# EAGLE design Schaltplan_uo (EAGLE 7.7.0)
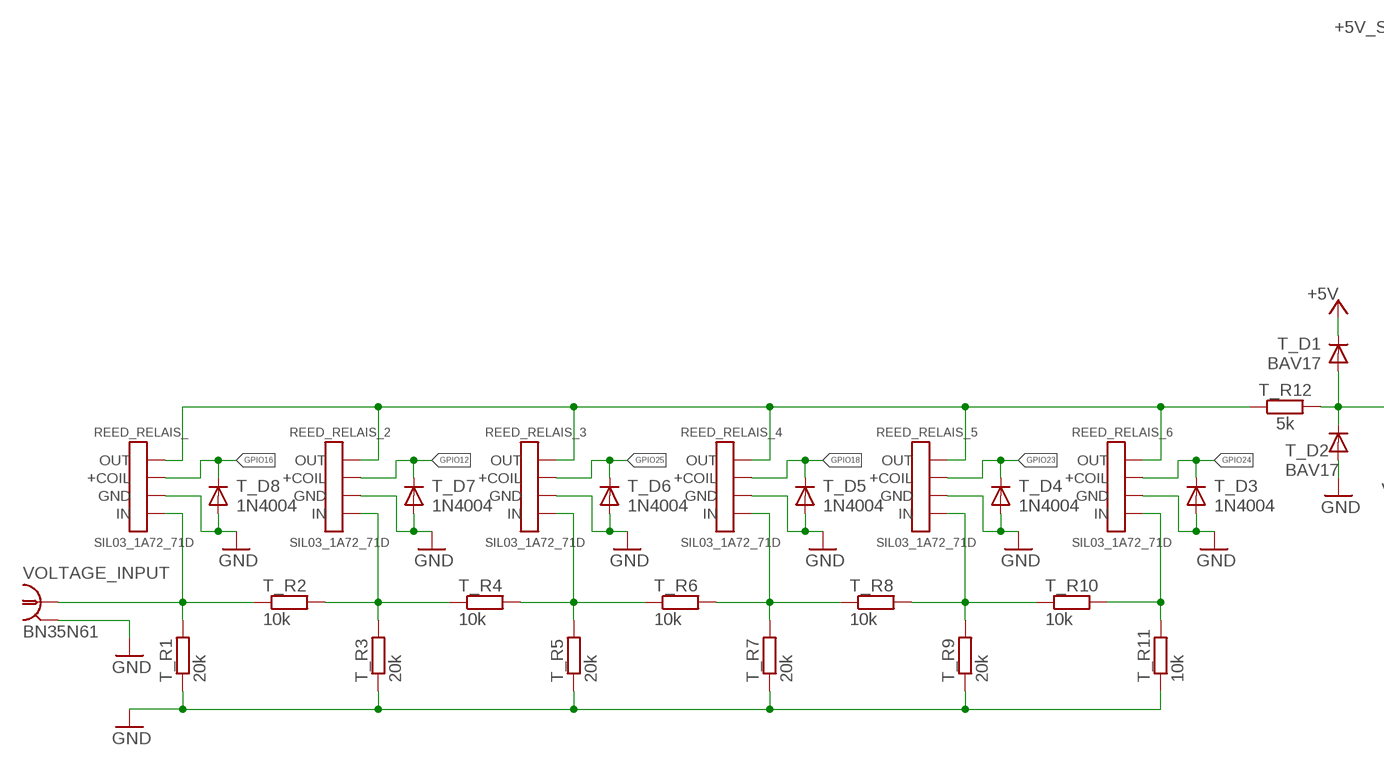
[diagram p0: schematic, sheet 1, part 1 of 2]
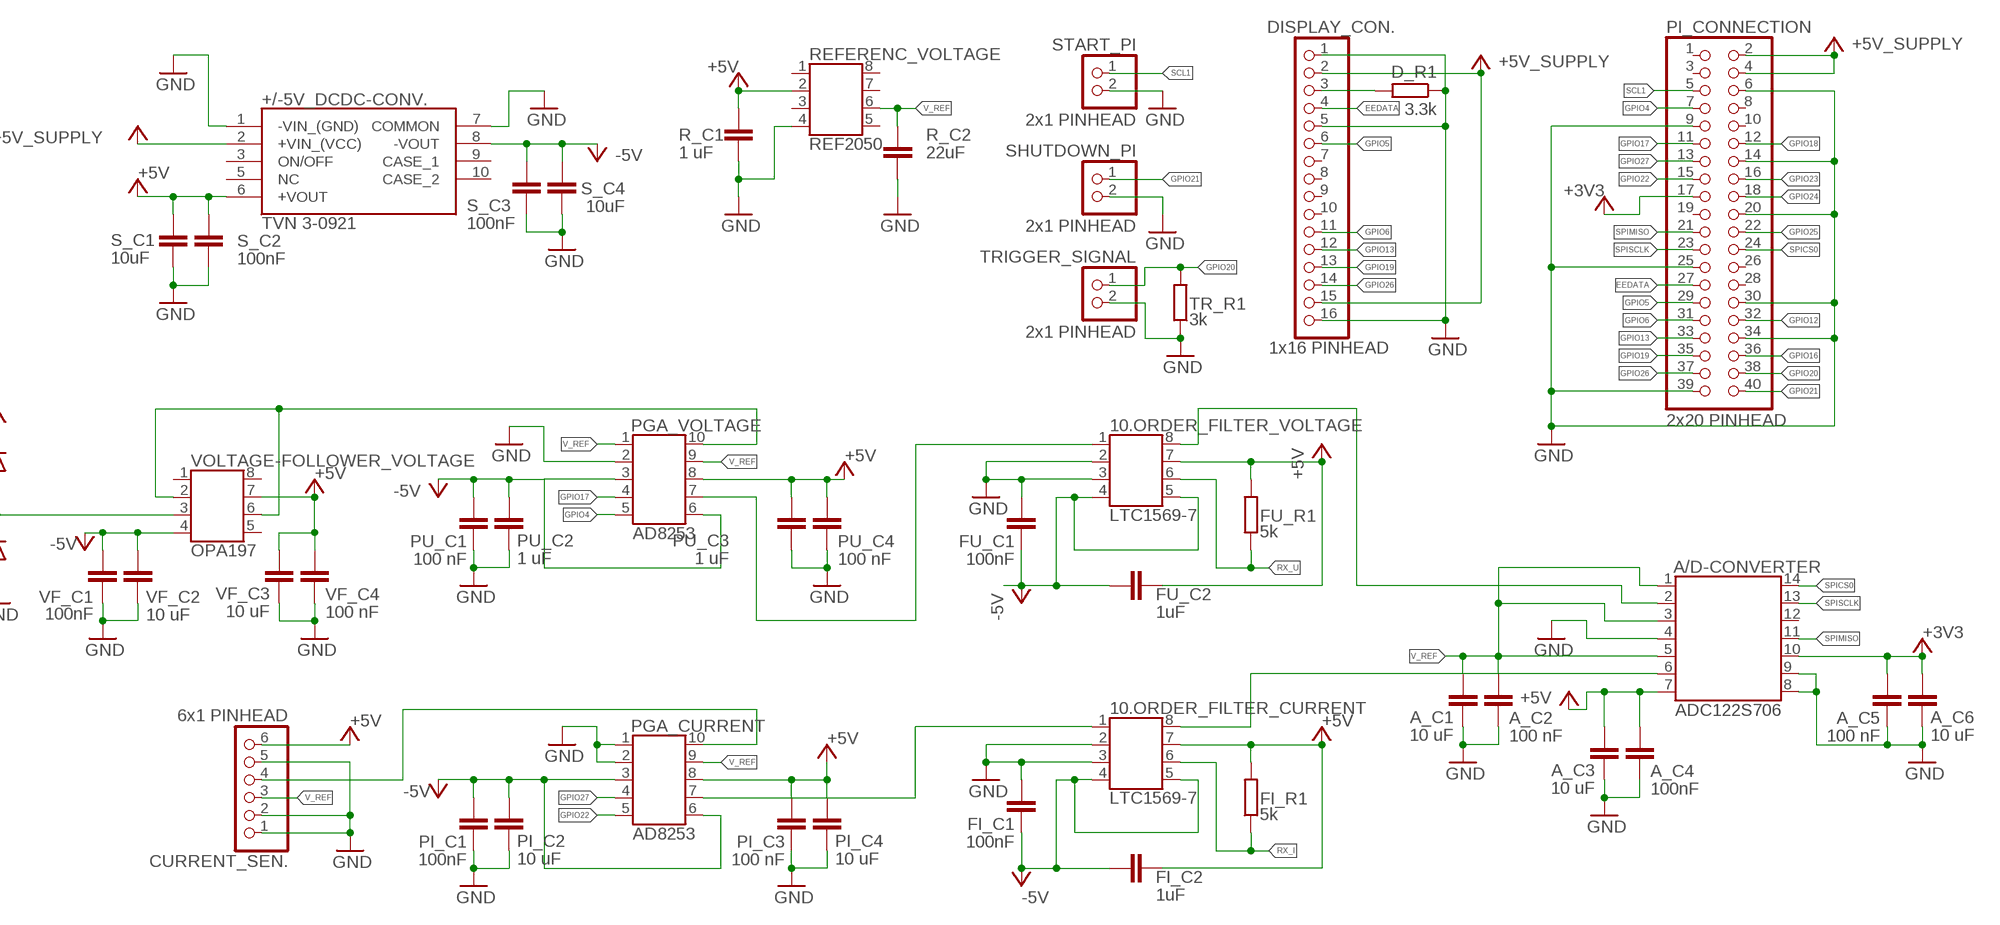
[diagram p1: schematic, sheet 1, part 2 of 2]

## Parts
10.ORDER_FILTER_CURRENT  LTC1569-7  SSOP8_TO_DIP8  [SSOP8_TO_DIP8]
10.ORDER_FILTER_VOLTAGE  LTC1569-7  SSOP8_TO_DIP8  [SSOP8_TO_DIP8]
+/-5V_DCDC-CONV.  TVN 3-0921  TVN_3-1223  [TVN32419]
A/D-CONVERTER  ADC122S706  SSOP14_TO_DIP14-6  [SSOP14_TO_DIP14-6]
A_C1  10 uF  C-EU025-030X050  [C025-030X050]
A_C2  100 nF  C-EU025-030X050  [C025-030X050]
A_C3  10 uF  C-EU025-030X050  [C025-030X050]
A_C4  100nF  C-EU025-030X050  [C025-030X050]
A_C5  100 nF  C-EU025-030X050  [C025-030X050]
A_C6  10 uF  C-EU025-030X050  [C025-030X050]
CURRENT_SEN.  6x1 PINHEAD  PINHD-1X6  [1X06]
D_R1  3.3k  R-EU_0207/10  [0207/10]
DISPLAY_CON.  1x16 PINHEAD  PINHD-1X16  [1X16]
FI_C1  100nF  C-EU025-030X050  [C025-030X050]
FI_C2  1uF  C-EU025-030X050  [C025-030X050]
FI_R1  5k  R-EU_0207/10  [0207/10]
FU_C1  100nF  C-EU025-030X050  [C025-030X050]
FU_C2  1uF  C-EU025-030X050  [C025-030X050]
FU_R1  5k  R-EU_0207/10  [0207/10]
PGA_CURRENT  AD8253  SSOP10_TO_DIP10  [SSOP10_TO_DIP10]
PGA_VOLTAGE  AD8253  SSOP10_TO_DIP10  [SSOP10_TO_DIP10]
PI_C1  100nF  C-EU025-030X050  [C025-030X050]
PI_C2  10 uF  C-EU025-030X050  [C025-030X050]
PI_C3  100 nF  C-EU025-030X050  [C025-030X050]
PI_C4  10 uF  C-EU025-030X050  [C025-030X050]
PI_CONNECTION  2x20 PINHEAD  PINHD-2X20  [2X20]
PU_C1  100 nF  C-EU025-030X050  [C025-030X050]
PU_C2  1 uF  C-EU025-030X050  [C025-030X050]
PU_C3  1 uF  C-EU025-030X050  [C025-030X050]
PU_C4  100 nF  C-EU025-030X050  [C025-030X050]
R_C1  1 uF  C-EU025-030X050  [C025-030X050]
R_C2  22uF  C-EU025-030X050  [C025-030X050]
REED_RELAIS_  SIL03_1A72_71D  REED_REALIS_SIL03_1A72_71D  [REED_RELAIS_SIL03_1A72_71D]
REED_RELAIS_2  SIL03_1A72_71D  REED_REALIS_SIL03_1A72_71D  [REED_RELAIS_SIL03_1A72_71D]
REED_RELAIS_3  SIL03_1A72_71D  REED_REALIS_SIL03_1A72_71D  [REED_RELAIS_SIL03_1A72_71D]
REED_RELAIS_4  SIL03_1A72_71D  REED_REALIS_SIL03_1A72_71D  [REED_RELAIS_SIL03_1A72_71D]
REED_RELAIS_5  SIL03_1A72_71D  REED_REALIS_SIL03_1A72_71D  [REED_RELAIS_SIL03_1A72_71D]
REED_RELAIS_6  SIL03_1A72_71D  REED_REALIS_SIL03_1A72_71D  [REED_RELAIS_SIL03_1A72_71D]
REFERENC_VOLTAGE  REF2050  SSOP8_TO_DIP8  [SSOP8_TO_DIP8]
S_C1  10uF  C-EU025-030X050  [C025-030X050]
S_C2  100nF  C-EU025-030X050  [C025-030X050]
S_C3  100nF  C-EU025-030X050  [C025-030X050]
S_C4  10uF  C-EU025-030X050  [C025-030X050]
SHUTDOWN_PI  2x1 PINHEAD  PINHD-1X2  [1X02]
START_PI  2x1 PINHEAD  PINHD-1X2  [1X02]
T_D1  BAV17  [DO35-10]
T_D2  BAV17  [DO35-10]
T_D3  1N4004  BAV17  [DO35-10]
T_D4  1N4004  BAV17  [DO35-10]
T_D5  1N4004  BAV17  [DO35-10]
T_D6  1N4004  BAV17  [DO35-10]
T_D7  1N4004  BAV17  [DO35-10]
T_D8  1N4004  BAV17  [DO35-10]
T_R1  20k  R-EU_0207/10  [0207/10]
T_R2  10k  R-EU_0207/10  [0207/10]
T_R3  20k  R-EU_0207/10  [0207/10]
T_R4  10k  R-EU_0207/10  [0207/10]
T_R5  20k  R-EU_0207/10  [0207/10]
T_R6  10k  R-EU_0207/10  [0207/10]
T_R7  20k  R-EU_0207/10  [0207/10]
T_R8  10k  R-EU_0207/10  [0207/10]
T_R9  20k  R-EU_0207/10  [0207/10]
T_R10  10k  R-EU_0207/10  [0207/10]
T_R11  10k  R-EU_0207/10  [0207/10]
T_R12  5k  R-EU_0207/10  [0207/10]
TR_R1  3k  R-EU_0207/10  [0207/10]
TRIGGER_SIGNAL  2x1 PINHEAD  PINHD-1X2  [1X02]
VF_C1  100nF  C-EU025-030X050  [C025-030X050]
VF_C2  10 uF  C-EU025-030X050  [C025-030X050]
VF_C3  10 uF  C-EU025-030X050  [C025-030X050]
VF_C4  100 nF  C-EU025-030X050  [C025-030X050]
VOLTAGE-FOLLOWER_VOLTAGE  OPA197  SSOP8_TO_DIP8  [SSOP8_TO_DIP8]
VOLTAGE_INPUT  BN35N61  [B35N61]

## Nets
+3V3: A/D-CONVERTER.10 A_C5.1 A_C6.1 PI_CONNECTION.17
+5V: 10.ORDER_FILTER_CURRENT.7 10.ORDER_FILTER_VOLTAGE.7 +/-5V_DCDC-CONV..6(+VOUT) A/D-CONVERTER.7 A_C3.1 A_C4.1 CURRENT_SEN..6 FI_C2.2 FI_R1.2 FU_C2.1 FU_R1.2 PGA_CURRENT.8 PGA_VOLTAGE.8 PI_C3.1 PI_C4.1 PU_C3.1 PU_C4.1 R_C1.1 REFERENC_VOLTAGE.2 S_C1.1 S_C2.1 T_D1.C VF_C3.1 VF_C4.1 VOLTAGE-FOLLOWER_VOLTAGE.7
+5V_SUPPLY: +/-5V_DCDC-CONV..2(+VIN_(VCC)) DISPLAY_CON..2 DISPLAY_CON..15 PI_CONNECTION.2 PI_CONNECTION.4
-5V: 10.ORDER_FILTER_CURRENT.4 10.ORDER_FILTER_CURRENT.5 10.ORDER_FILTER_VOLTAGE.4 10.ORDER_FILTER_VOLTAGE.5 +/-5V_DCDC-CONV..8(-VOUT) FI_C1.1 FI_C2.1 FU_C1.1 FU_C2.2 PGA_CURRENT.3 PGA_CURRENT.6 PGA_VOLTAGE.3 PGA_VOLTAGE.6 PI_C1.1 PI_C2.2 PU_C1.1 PU_C2.2 S_C3.1 S_C4.2 VF_C1.1 VF_C2.2 VOLTAGE-FOLLOWER_VOLTAGE.4
EEDATA: DISPLAY_CON..4 PI_CONNECTION.27
GND: 10.ORDER_FILTER_CURRENT.2 10.ORDER_FILTER_CURRENT.3 10.ORDER_FILTER_VOLTAGE.2 10.ORDER_FILTER_VOLTAGE.3 +/-5V_DCDC-CONV..1(-VIN_(GND)) +/-5V_DCDC-CONV..7(COMMON) A/D-CONVERTER.4 A/D-CONVERTER.8 A/D-CONVERTER.9 A_C1.2 A_C2.2 A_C3.2 A_C4.2 A_C5.2 A_C6.2 CURRENT_SEN..1 CURRENT_SEN..2 CURRENT_SEN..5 D_R1.1 DISPLAY_CON..1 DISPLAY_CON..5 DISPLAY_CON..16 FI_C1.2 FU_C1.2 PGA_CURRENT.1 PGA_CURRENT.2 PGA_VOLTAGE.2 PI_C1.2 PI_C2.1 PI_C3.2 PI_C4.2 PI_CONNECTION.6 PI_CONNECTION.9 PI_CONNECTION.14 PI_CONNECTION.20 PI_CONNECTION.25 PI_CONNECTION.30 PI_CONNECTION.34 PI_CONNECTION.39 PU_C1.2 PU_C2.1 PU_C3.2 PU_C4.2 R_C1.2 R_C2.2 REED_RELAIS_2.P$3(GND) REED_RELAIS_3.P$3(GND) REED_RELAIS_4.P$3(GND) REED_RELAIS_5.P$3(GND) REED_RELAIS_6.P$3(GND) REED_RELAIS_.P$3(GND) REFERENC_VOLTAGE.4 S_C1.2 S_C2.2 S_C3.2 S_C4.1 SHUTDOWN_PI.2 START_PI.2 T_D2.A T_D3.A T_D4.A T_D5.A T_D6.A T_D7.A T_D8.A T_R1.1 T_R3.1 T_R5.1 T_R7.1 T_R9.1 T_R11.1 TR_R1.1 TRIGGER_SIGNAL.2 VF_C1.2 VF_C2.1 VF_C3.2 VF_C4.2 VOLTAGE_INPUT.2 VOLTAGE_INPUT.3 VOLTAGE_INPUT.4 VOLTAGE_INPUT.5
GPIO4: PGA_VOLTAGE.5 PI_CONNECTION.7
GPIO5: DISPLAY_CON..6 PI_CONNECTION.29
GPIO6: DISPLAY_CON..11 PI_CONNECTION.31
GPIO12: PI_CONNECTION.32 REED_RELAIS_2.P$2(+COIL) T_D7.C
GPIO13: DISPLAY_CON..12 PI_CONNECTION.33
GPIO16: PI_CONNECTION.36 REED_RELAIS_.P$2(+COIL) T_D8.C
GPIO17: PGA_VOLTAGE.4 PI_CONNECTION.11
GPIO18: PI_CONNECTION.12 REED_RELAIS_4.P$2(+COIL) T_D5.C
GPIO19: DISPLAY_CON..13 PI_CONNECTION.35
GPIO20: PI_CONNECTION.38 TR_R1.2 TRIGGER_SIGNAL.1
GPIO21: PI_CONNECTION.40 SHUTDOWN_PI.1
GPIO22: PGA_CURRENT.5 PI_CONNECTION.15
GPIO23: PI_CONNECTION.16 REED_RELAIS_5.P$2(+COIL) T_D4.C
GPIO24: PI_CONNECTION.18 REED_RELAIS_6.P$2(+COIL) T_D3.C
GPIO25: PI_CONNECTION.22 REED_RELAIS_3.P$2(+COIL) T_D6.C
GPIO26: DISPLAY_CON..14 PI_CONNECTION.37
GPIO27: PGA_CURRENT.4 PI_CONNECTION.13
N$2: REED_RELAIS_2.P$1(OUT) REED_RELAIS_3.P$1(OUT) REED_RELAIS_4.P$1(OUT) REED_RELAIS_5.P$1(OUT) REED_RELAIS_6.P$1(OUT) REED_RELAIS_.P$1(OUT) T_R12.1
N$3: D_R1.2 DISPLAY_CON..3
N$42: REED_RELAIS_2.P$4(IN) T_R2.2 T_R3.2 T_R4.1
N$43: REED_RELAIS_3.P$4(IN) T_R4.2 T_R5.2 T_R6.1
N$44: REED_RELAIS_4.P$4(IN) T_R6.2 T_R7.2 T_R8.1
N$45: REED_RELAIS_5.P$4(IN) T_R8.2 T_R9.2 T_R10.1
N$46: REED_RELAIS_6.P$4(IN) T_R10.2 T_R11.2
RX_I: 10.ORDER_FILTER_CURRENT.6 FI_R1.1
RX_U: 10.ORDER_FILTER_VOLTAGE.6 FU_R1.1
SCL1: PI_CONNECTION.5 START_PI.1
SIGNAL_I_2: CURRENT_SEN..4 PGA_CURRENT.10
SIGNAL_I_3: 10.ORDER_FILTER_CURRENT.1 PGA_CURRENT.7
SIGNAL_I_4: 10.ORDER_FILTER_CURRENT.8 A/D-CONVERTER.6
SIGNAL_U_0: REED_RELAIS_.P$4(IN) T_R1.2 T_R2.1 VOLTAGE_INPUT.1
SIGNAL_U_1: T_D1.A T_D2.C T_R12.2 VOLTAGE-FOLLOWER_VOLTAGE.3
SIGNAL_U_2: PGA_VOLTAGE.10 VOLTAGE-FOLLOWER_VOLTAGE.2 VOLTAGE-FOLLOWER_VOLTAGE.6
SIGNAL_U_3: 10.ORDER_FILTER_VOLTAGE.1 PGA_VOLTAGE.7
SIGNAL_U_4: 10.ORDER_FILTER_VOLTAGE.8 A/D-CONVERTER.2
SPICS0: A/D-CONVERTER.14 PI_CONNECTION.24
SPIMISO: A/D-CONVERTER.11 PI_CONNECTION.21
SPISCLK: A/D-CONVERTER.13 PI_CONNECTION.23
V_REF: A/D-CONVERTER.1 A/D-CONVERTER.3 A/D-CONVERTER.5 A_C1.1 A_C2.1 CURRENT_SEN..3 PGA_CURRENT.9 PGA_VOLTAGE.1 PGA_VOLTAGE.9 R_C2.1 REFERENC_VOLTAGE.6
Unconnected: +/-5V_DCDC-CONV..3(ON/OFF) +/-5V_DCDC-CONV..5(NC) +/-5V_DCDC-CONV..9(CASE_1) +/-5V_DCDC-CONV..10(CASE_2) A/D-CONVERTER.12 DISPLAY_CON..7 DISPLAY_CON..8 DISPLAY_CON..9 DISPLAY_CON..10 PI_CONNECTION.1 PI_CONNECTION.3 PI_CONNECTION.8 PI_CONNECTION.10 PI_CONNECTION.19 PI_CONNECTION.26 PI_CONNECTION.28 REFERENC_VOLTAGE.1 REFERENC_VOLTAGE.3 REFERENC_VOLTAGE.5 REFERENC_VOLTAGE.7 REFERENC_VOLTAGE.8 VOLTAGE-FOLLOWER_VOLTAGE.1 VOLTAGE-FOLLOWER_VOLTAGE.5 VOLTAGE-FOLLOWER_VOLTAGE.8

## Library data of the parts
10.ORDER_FILTER_CURRENT 10.ORDER_FILTER_VOLTAGE REFERENC_VOLTAGE VOLTAGE-FOLLOWER_VOLTAGE = OWN_Library:SSOP8_TO_DIP8
+/-5V_DCDC-CONV. = TVN_3-1223:TVN_3-1223: Isolated DC/DC Converters 3W 9-18Vin SIP-8 +/-15Vout +/-100mA Source: Datasheet; ALLIED_NUMBER: 71099550; ALLIED_PRICE-STOCK: https://www.alliedelec.com/traco-power-tvn-3-1223/71099550/; DESCRIPTION: Isolated DC/DC Converters 3W 9-18Vin SIP-8 +/-15Vout +/-100mA; HEIGHT: 11mm; MANUFACTURER_NAME: Traco Power; MANUFACTURER_PART_NUMBER: TVN 3-1223; MOUSER_PART_NUMBER: 495-TVN3-1223; MOUSER_PRICE-STOCK: https://www.mouser.com/Search/Refine.aspx?Keyword=495-TVN3-1223; RS_PART_NUMBER: 1466094; RS_PRICE-STOCK: https://uk.rs-online.com/web/p/products/1466094
A/D-CONVERTER = OWN_Library:SSOP14_TO_DIP14-6: SSOP14 SMD to DIP14-6 ADAPTER
A_C1-A_C6 FI_C1 FI_C2 FU_C1 FU_C2 PI_C1-PI_C4 PU_C1-PU_C4 R_C1 R_C2 S_C1-S_C4 VF_C1-VF_C4 = rcl:C-EU: CAPACITOR, European symbol
CURRENT_SEN. = pinhead:PINHD-1X6: PIN HEADER
D_R1 FI_R1 FU_R1 T_R1-T_R12 TR_R1 = rcl:R-EU_: RESISTOR, European symbol
DISPLAY_CON. = pinhead:PINHD-1X16: PIN HEADER
PGA_CURRENT PGA_VOLTAGE = OWN_Library:SSOP10_TO_DIP10
PI_CONNECTION = pinhead:PINHD-2X20: PIN HEADER
REED_RELAIS_ REED_RELAIS_2-REED_RELAIS_6 = OWN_Library:REED_REALIS_SIL03_1A72_71D
SHUTDOWN_PI START_PI TRIGGER_SIGNAL = pinhead:PINHD-1X2: PIN HEADER
T_D1-T_D8 = diode:BAV17: DIODE
VOLTAGE_INPUT = con-coax:BN35N61: BNC CONNECTOR; OC_FARNELL: unknown; OC_NEWARK: unknown

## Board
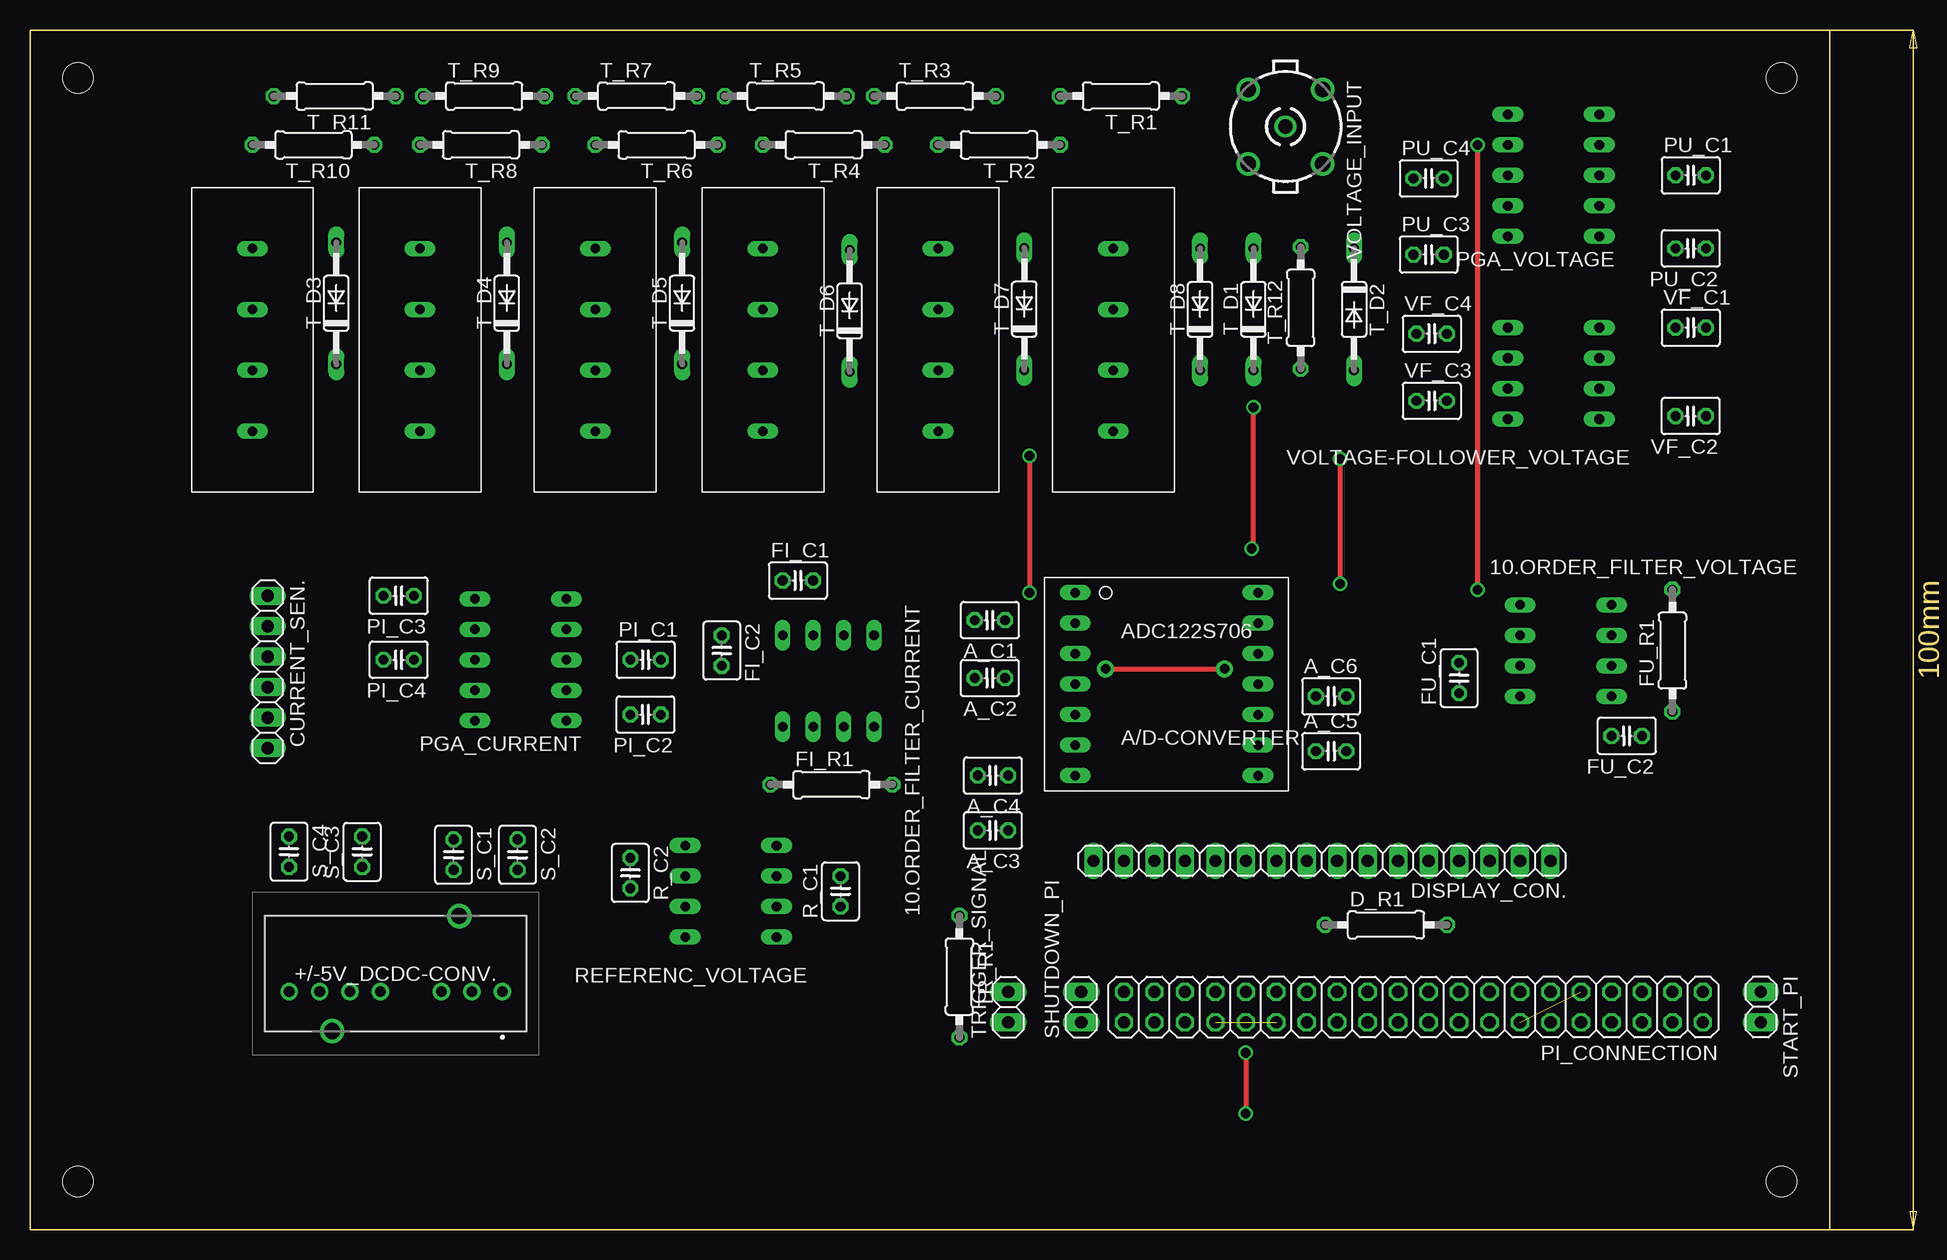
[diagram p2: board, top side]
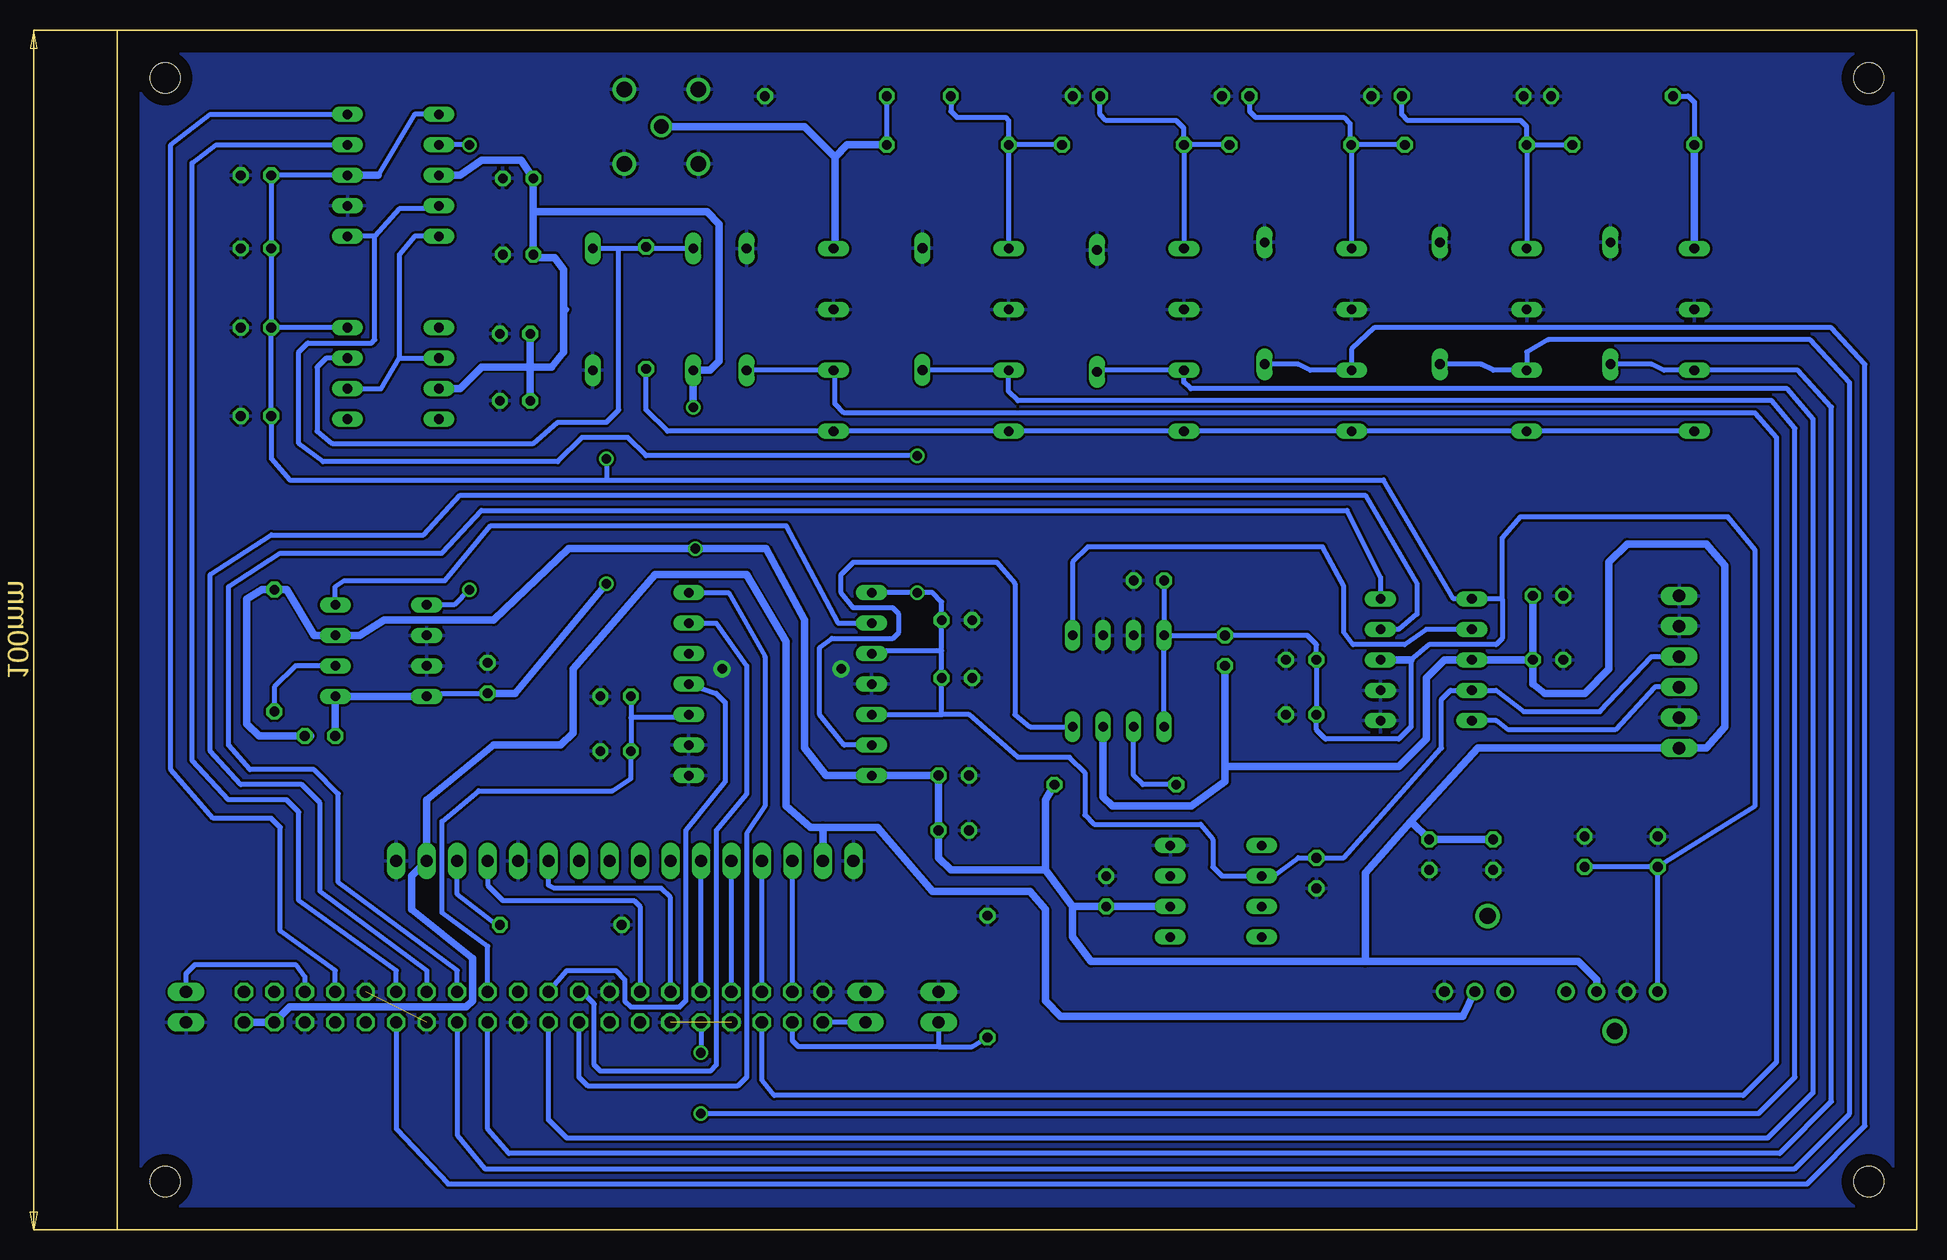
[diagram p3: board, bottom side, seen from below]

Size 157.27 x 100 mm. Coordinates in mm from the lower left corner, seen from the top.
Outline: 0,0 0,100 150,100 150,0 0,0
Copper layers (1*16): Top 0.035mm / dielectric 1.5mm / Bottom 0.035mm
Design rules "default": minimum track width 10mil, minimum drill 24mil, track to track 8mil, track to pad 8mil, pad to pad 8mil, via to via 8mil, smd to smd 8mil, copper to edge 40mil, drill to drill 8mil, minimum pad ring 10mil, minimum via ring 8mil, stop-mask expansion 4mil, vias tented up to drill 0mil, thermal gap 10mil
Holes 2.5 mm at 4,96 146,96 146,4 4,4

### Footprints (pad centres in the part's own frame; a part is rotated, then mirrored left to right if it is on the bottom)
SSOP8_TO_DIP8 = drill 0.8 long: 1 -5.08,2.54; 2 -5.08,0; 3 -5.08,-2.54; 4 -5.08,-5.08; 5 2.54,-5.08; 6 2.54,-2.54; 7 2.54,0; 8 2.54,2.54
TVN32419 = drill 0.89 pad 1.446: 1 -8.9,1.5; 2 -6.36,1.5; 3 -3.82,1.5; 5 1.26,1.5; 6 3.8,1.5; 7 6.34,1.5; 8 8.88,1.5 | drill 1.35 pad 2.025: 9 -5.3,-4.8; 10 5.3,4.8
SSOP14_TO_DIP14-6 = drill 0.8 long: 1 -7.62,7.62; 2 -7.62,5.08; 3 -7.62,2.54; 4 -7.62,0; 5 -7.62,-2.54; 6 -7.62,-5.08; 7 -7.62,-7.62; 8 7.62,-7.62; 9 7.62,-5.08; 10 7.62,-2.54; 11 7.62,0; 12 7.62,2.54; 13 7.62,5.08; 14 7.62,7.62
C025-030X050 = drill 0.813 octagon: 1 -1.27,0; 2 1.27,0
1X06 = drill 1.016 long: 1 -6.35,0; 2 -3.81,0; 3 -1.27,0; 4 1.27,0; 5 3.81,0; 6 6.35,0
0207/10 = drill 0.813 octagon: 1 -5.08,0; 2 5.08,0
1X16 = drill 1.016 long: 1 -19.05,0; 2 -16.51,0; 3 -13.97,0; 4 -11.43,0; 5 -8.89,0; 6 -6.35,0; 7 -3.81,0; 8 -1.27,0; 9 1.27,0; 10 3.81,0; 11 6.35,0; 12 8.89,0; 13 11.43,0; 14 13.97,0; 15 16.51,0; 16 19.05,0
SSOP10_TO_DIP10 = drill 0.8 long: 1 -2.54,2.54; 2 -2.54,0; 3 -2.54,-2.54; 4 -2.54,-5.08; 5 -2.54,-7.62; 6 5.08,-7.62; 7 5.08,-5.08; 8 5.08,-2.54; 9 5.08,0; 10 5.08,2.54
2X20 = drill 1.016 octagon: 1 -24.13,-1.27; 2 -24.13,1.27; 3 -21.59,-1.27; 4 -21.59,1.27; 5 -19.05,-1.27; 6 -19.05,1.27; 7 -16.51,-1.27; 8 -16.51,1.27; 9 -13.97,-1.27; 10 -13.97,1.27; 11 -11.43,-1.27; 12 -11.43,1.27; 13 -8.89,-1.27; 14 -8.89,1.27; 15 -6.35,-1.27; 16 -6.35,1.27; 17 -3.81,-1.27; 18 -3.81,1.27; 19 -1.27,-1.27; 20 -1.27,1.27; 21 1.27,-1.27; 22 1.27,1.27; 23 3.81,-1.27; 24 3.81,1.27; 25 6.35,-1.27; 26 6.35,1.27; 27 8.89,-1.27; 28 8.89,1.27; 29 11.43,-1.27; 30 11.43,1.27; 31 13.97,-1.27; 32 13.97,1.27; 33 16.51,-1.27; 34 16.51,1.27; 35 19.05,-1.27; 36 19.05,1.27; 37 21.59,-1.27; 38 21.59,1.27; 39 24.13,-1.27; 40 24.13,1.27
REED_RELAIS_SIL03_1A72_71D = drill 0.8 long: P$1 0,0; P$2 0,-5.08; P$3 0,-10.16; P$4 0,-15.24
1X02 = drill 1.016 long: 1 -1.27,0; 2 1.27,0
DO35-10 = drill 0.813 long: A 5.08,0; C -5.08,0
B35N61 = drill 1.2: 1 0,0 | drill 1.3: 2 3.099,3.099; 3 -3.099,3.099; 4 -3.099,-3.099; 5 3.099,-3.099

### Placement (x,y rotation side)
10.ORDER_FILTER_CURRENT  67.82,44.45 270 top
10.ORDER_FILTER_VOLTAGE  129.29,49.53 0 top
+/-5V_DCDC-CONV.  30.48,21.34 180 top
A/D-CONVERTER  94.74,45.47 0 top
A_C1  80.01,50.8 180 top
A_C2  80.01,45.97 180 top
A_C3  80.26,33.27 180 top
A_C4  80.26,37.85 180 top
A_C5  108.46,39.88 0 top
A_C6  108.46,44.45 0 top
CURRENT_SEN.  19.81,46.48 270 top
D_R1  113.03,25.4 0 top
DISPLAY_CON.  107.7,30.73 180 top
FI_C1  64.01,54.1 0 top
FI_C2  57.66,48.26 270 top
FI_R1  66.8,37.08 0 top
FU_C1  119.13,45.97 90 top
FU_C2  133.1,41.15 180 top
FU_R1  136.91,48.26 90 top
PGA_CURRENT  42.16,44.96 180 top
PGA_VOLTAGE  128.27,85.34 180 top
PI_C1  51.31,47.5 0 top
PI_C2  51.31,42.93 180 top
PI_C3  30.73,52.83 180 top
PI_C4  30.73,47.5 180 top
PI_CONNECTION  115.32,18.54 180 top
PU_C1  138.43,87.88 0 top
PU_C2  138.43,81.79 180 top
PU_C3  116.59,81.28 0 top
PU_C4  116.59,87.63 0 top
R_C1  67.56,28.19 90 top
R_C2  50.04,29.72 270 top
REED_RELAIS_  90.3,66.55 180 top
REED_RELAIS_2  75.69,66.55 180 top
REED_RELAIS_3  61.09,66.55 180 top
REED_RELAIS_4  47.12,66.55 180 top
REED_RELAIS_5  32.51,66.55 180 top
REED_RELAIS_6  18.54,66.55 180 top
REFERENC_VOLTAGE  57.15,26.92 180 top
S_C1  35.31,31.24 270 top
S_C2  40.64,31.24 270 top
S_C3  27.69,31.5 90 top
S_C4  21.59,31.5 270 top
SHUTDOWN_PI  87.63,18.54 90 top
START_PI  144.27,18.54 270 top
T_D1  101.98,76.71 90 top
T_D2  110.36,76.71 270 top
T_D3  25.53,77.22 90 top
T_D4  39.75,77.22 90 top
T_D5  54.36,77.22 90 top
T_D6  68.33,76.58 90 top
T_D7  82.88,76.73 90 top
T_D8  97.54,76.71 90 top
T_R1  90.93,94.49 180 top
T_R2  80.77,90.42 180 top
T_R3  75.44,94.49 0 top
T_R4  66.17,90.42 180 top
T_R5  62.99,94.49 0 top
T_R6  52.22,90.42 180 top
T_R7  50.55,94.49 0 top
T_R8  37.59,90.42 180 top
T_R9  37.85,94.49 0 top
T_R10  23.62,90.42 180 top
T_R11  25.4,94.49 180 top
T_R12  105.92,76.83 90 top
TR_R1  77.47,21.08 270 top
TRIGGER_SIGNAL  81.53,18.54 90 top
VF_C1  138.43,75.18 0 top
VF_C2  138.43,67.82 180 top
VF_C3  116.84,69.09 0 top
VF_C4  116.84,74.68 0 top
VOLTAGE-FOLLOWER_VOLTAGE  125.73,70.1 180 top
VOLTAGE_INPUT  104.65,91.95 270 top

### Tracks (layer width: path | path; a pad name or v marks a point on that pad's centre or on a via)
+3V3
  Bottom 0.406: A_C6.1 107.19,42.67 | 107.19,42.67 A_C5.1 107.19,37.59 108.71,36.58 119.89,36.58 122.94,34.04 122.94,26.42 119.13,23.62 PI_CONNECTION.17 | A/D-CONVERTER.10 102.62,42.67 107.19,42.67
+5V  (via drill 0.8)
  Top 0.406: v101.83,56.77 101.98,56.77 v101.98,68.53
  Bottom 0.406: 115.06,81.03 PU_C3.1 | v101.98,68.53 101.88,68.43 | 112.52,76.71 112.78,76.45
  Bottom 0.61: 133.86,41.15 FU_C2.1 138.18,41.15 139.19,42.16 139.19,52.58 137.92,53.34 FU_R1.2 135.89,53.34 133.6,49.53 10.ORDER_FILTER_VOLTAGE.7 129.79,49.53 127.76,50.8 118.62,50.8 112.39,56.77 v101.83,56.77 95.94,56.77 92.71,50.8 92.71,40.13 90.93,37.85 A/D-CONVERTER.7 A_C4.1 A_C3.1 81.53,30.99 80.52,29.97 72.64,29.97 | PI_C4.1 32,45.47 30.99,44.7 27.69,44.7 25.65,46.74 25.65,55.63 24.13,57.15 17.53,57.15 16,55.37 16,41.91 17.53,40.13 CURRENT_SEN..6 36.58,40.13 42.16,34.04 | PI_C3.1 PI_C4.1 | PI_C4.1 PGA_CURRENT.8 39.37,47.5 40.89,45.97 40.89,40.89 43.18,38.61 57.66,38.61 | 42.16,34.04 45.97,29.72 45.97,22.35 | FI_R1.2 72.64,35.81 72.64,29.97 | 45.97,22.35 28.23,22.35 26.68,20.8 +/-5V_DCDC-CONV..6 | 45.97,22.35 68.83,22.35 70.36,24.38 70.36,26.92 | 72.64,29.97 70.36,26.92 | 115.57,71.88 VF_C4.1 | 115.57,71.88 119.63,71.88 121.41,70.1 VOLTAGE-FOLLOWER_VOLTAGE.7 | VF_C3.1 115.57,71.88 | 115.57,71.88 113.79,71.88 112.78,73.15 112.78,76.45 112.78,80.01 113.54,81.03 115.06,81.03 | 115.32,84.84 PU_C4.1 116.33,89.15 119.63,89.15 121.41,87.88 PGA_VOLTAGE.8 | 115.32,84.84 PU_C3.1 | FI_C2.2 57.66,38.61 | 57.66,38.61 57.66,37.34 60.45,35.31 67.06,35.31 67.82,36.07 10.ORDER_FILTER_CURRENT.7 | REFERENC_VOLTAGE.2 R_C1.1 70.36,26.92 | v101.98,68.53 T_D1.C 100.58,71.63 99.82,72.39 99.82,83.82 100.84,84.84 115.32,84.84 | S_C1.1 S_C2.1 42.16,34.04
+5V_SUPPLY
  Bottom 0.61: PI_CONNECTION.2 PI_CONNECTION.4 135.64,18.54 120.9,18.54 120.4,19.05 120.4,22.61 125.48,26.67 125.48,29.46 DISPLAY_CON..2 124.21,35.81 118.62,40.39 113.03,40.39 112.01,41.4 112.01,46.74 105.16,54.61 97.54,54.61 94.23,49.02 94.23,35.31 92.2,33.53 91.19,33.53 | 91.19,33.53 86.61,33.53 82.04,28.19 73.91,28.19 72.64,26.67 72.64,19.05 71.37,17.78 37.85,17.78 +/-5V_DCDC-CONV..2 | DISPLAY_CON..15 91.19,33.53
-5V  (via drill 0.8)
  Top 0.406: v109.22,53.85 v109.22,64.26
  Bottom 0.406: 10.ORDER_FILTER_VOLTAGE.4 123.95,44.7 FU_C1.1 | 10.ORDER_FILTER_CURRENT.4 FI_C2.1 50.8,49.53 50.04,48.77 PI_C1.1 PI_C2.2 50.04,41.66 49.28,40.89 43.18,40.89 42.16,41.91 42.16,47.5 40.64,48.77 35.05,48.77 34.54,49.28 34.54,52.58 | 21.61,30.23 21.6,30.22 +/-5V_DCDC-CONV..8 | 21.61,30.23 S_C3.1 | 34.54,52.58 34.54,57.66 33.02,59.44 15.75,59.44 13.46,56.64 13.46,35.33 21.61,30.23 | 109.22,62.48 44.45,62.48 38.61,52.58 PGA_CURRENT.6 34.54,52.58 | PGA_VOLTAGE.6 125.22,92.96 128.27,87.88 | PGA_VOLTAGE.3 PU_C1.1 PU_C2.2 VF_C1.1 | VF_C1.1 VF_C2.2 137.16,64.26 135.64,62.48 109.22,62.48 | VOLTAGE-FOLLOWER_VOLTAGE.4 VF_C1.1 | 10.ORDER_FILTER_CURRENT.5 10.ORDER_FILTER_CURRENT.4 | FI_C1.1 10.ORDER_FILTER_CURRENT.4 | v109.22,64.26 109.22,62.48
  Bottom 0.61: FU_C2.2 10.ORDER_FILTER_VOLTAGE.5 10.ORDER_FILTER_VOLTAGE.4 | PGA_CURRENT.3 42.16,47.5 | FU_C1.1 116.84,44.7 v109.22,53.85 | 128.27,87.88 PGA_VOLTAGE.3 | 21.6,30.22 S_C4.2
EEDATA
  Bottom 0.406: DISPLAY_CON..4 119.13,28.7 117.86,27.43 106.93,27.43 106.43,26.92 PI_CONNECTION.27
GND  (via drill 0.8 pad 1.42)  (2 unrouted)
  Top 0.406: v89.66,46.74 v99.57,46.74
  Bottom 0.254: 124.08,17.21 PI_CONNECTION.14
  Bottom 0.406: v99.57,46.74 99.57,46.48
  pour Bottom: 2,2 2,98 148,98 148,2
GPIO4
  Bottom 0.406: PI_CONNECTION.7 131.83,21.59 136.4,24.89 136.4,33.53 137.16,34.29 141.99,34.29 145.54,38.35 145.54,90.42 142.24,92.96 PGA_VOLTAGE.5
GPIO5
  Bottom 0.406: PI_CONNECTION.29 103.89,27.69 104.65,28.45 113.54,28.45 114.05,28.7 DISPLAY_CON..6
GPIO6
  Bottom 0.406: PI_CONNECTION.31 DISPLAY_CON..11
GPIO12  (via drill 0.8)
  Top 0.406: v101.35,14.73 v101.35,9.65
  Bottom 0.406: v101.35,9.65 13.21,9.65 10.16,12.7 10.16,66.8 12.06,69.09 74.93,69.09 75.69,69.85 REED_RELAIS_2.P$2 77.7,71.65 T_D7.C | PI_CONNECTION.32 v101.35,14.73
GPIO13
  Bottom 0.406: PI_CONNECTION.33 DISPLAY_CON..12
GPIO16
  Bottom 0.406: PI_CONNECTION.36 96.27,12.45 95.25,11.18 14.48,11.18 11.68,13.97 11.68,66.04 13.46,68.07 89.41,68.07 90.17,68.83 90.17,71.5 REED_RELAIS_.P$2 T_D8.C
GPIO17
  Bottom 0.406: PGA_VOLTAGE.4 141.73,90.42 143.76,88.9 143.76,39.12 140.72,35.81 135.89,35.81 134.87,34.8 134.87,27.43 126.75,21.59 PI_CONNECTION.11
GPIO18
  Bottom 0.406: PI_CONNECTION.12 126.75,8.38 122.43,3.81 9.14,3.81 4.32,8.64 4.32,72.14 7.11,75.18 45.21,75.18 47.12,73.38 REED_RELAIS_4.P$2 50.55,71.63 51.56,72.14 T_D5.C
GPIO19
  Bottom 0.406: PI_CONNECTION.35 DISPLAY_CON..13
GPIO20
  Bottom 0.406: 81.53,15.24 93.22,15.24 93.73,15.75 PI_CONNECTION.38 | TRIGGER_SIGNAL.1 81.53,15.24 | 81.53,15.24 78.74,15.24 TR_R1.2
GPIO21
  Bottom 0.406: SHUTDOWN_PI.1 PI_CONNECTION.40
GPIO22
  Bottom 0.406: PGA_CURRENT.5 44.7,54.36 47.5,59.94 119.63,59.94 122.94,56.39 136.4,56.39 140.72,53.59 140.72,40.39 138.94,38.35 133.6,38.35 131.57,36.32 131.57,28.96 121.67,21.59 PI_CONNECTION.15
GPIO23
  Bottom 0.406: PI_CONNECTION.16 121.67,7.87 119.38,5.08 10.16,5.08 5.59,9.65 5.59,70.61 8.89,74.17 30.73,74.17 32.51,73.15 REED_RELAIS_5.P$2 35.31,71.63 36.32,72.14 T_D4.C
GPIO24
  Bottom 0.406: PI_CONNECTION.18 119.13,8.38 117.35,6.35 11.43,6.35 7.11,10.67 7.11,68.58 9.91,71.63 REED_RELAIS_6.P$2 21.08,71.63 22.1,72.14 T_D3.C
GPIO25
  Bottom 0.406: PI_CONNECTION.22 114.3,17.02 114.05,16.76 114.05,9.14 112.52,7.62 12.45,7.62 8.64,11.43 8.64,67.56 10.79,70.1 60.5,70.1 61.09,70.64 REED_RELAIS_3.P$2 68.38,71.63 T_D6.C
GPIO26
  Bottom 0.406: PI_CONNECTION.37 DISPLAY_CON..14
GPIO27
  Bottom 0.406: PGA_CURRENT.4 43.18,50.04 41.66,51.31 41.66,53.85 45.97,61.21 121.41,61.21 124.46,57.91 137.16,57.91 142.24,54.61 142.24,39.88 139.7,37.08 134.62,37.08 133.1,35.56 133.1,28.19 124.21,21.59 PI_CONNECTION.13
N$2
  Bottom 0.406: REED_RELAIS_6.P$1 REED_RELAIS_5.P$1 REED_RELAIS_4.P$1 REED_RELAIS_3.P$1 REED_RELAIS_2.P$1 REED_RELAIS_.P$1 104.14,66.55 105.92,68.33 T_R12.1
N$3
  Bottom 0.406: D_R1.2 118.36,25.4 121.67,27.94 DISPLAY_CON..3
N$42
  Bottom 0.406: T_R4.1 T_R2.2 | T_R3.2 80.52,93.22 80.01,92.71 75.95,92.71 75.69,92.46 T_R2.2 | T_R2.2 REED_RELAIS_2.P$4
N$43
  Bottom 0.406: 61.06,81.81 REED_RELAIS_3.P$4 T_R4.2 | T_R6.1 T_R4.2 | T_R4.2 61.09,91.82 61.72,92.46 67.56,92.46 68.07,92.96 T_R5.2
N$44
  Bottom 0.406: 42.42,90.42 T_R8.1 T_R6.2 | T_R6.2 47.14,81.81 REED_RELAIS_4.P$4 | T_R7.2 55.63,93.22 55.12,92.71 47.75,92.71 47.24,92.2 47.24,90.53 T_R6.2
N$45
  Bottom 0.406: T_R8.2 T_R10.1 | T_R8.2 REED_RELAIS_5.P$4 | T_R8.2 32.51,91.95 33.02,92.46 42.42,92.46 42.93,92.96 T_R9.2
N$46
  Bottom 0.406: T_R11.2 19.05,94.49 18.54,93.98 T_R10.2
  Bottom 0.61: T_R10.2 REED_RELAIS_6.P$4
RX_I
  Bottom 0.406: FI_R1.1 64.52,37.08 65.28,37.85 10.ORDER_FILTER_CURRENT.6
RX_U
  Bottom 0.406: 10.ORDER_FILTER_VOLTAGE.6 135.13,46.99 136.91,45.21 FU_R1.1
SCL1
  Bottom 0.406: START_PI.1 144.27,21.34 143.51,22.1 135.13,22.1 134.37,21.08 PI_CONNECTION.5
SIGNAL_I_2
  Bottom 0.406: CURRENT_SEN..4 21.84,45.21 25.15,41.66 34.04,41.66 35.05,42.42 PGA_CURRENT.10
SIGNAL_I_3
  Bottom 0.406: PGA_CURRENT.7 40.89,50.04 42.67,48.77 46.99,48.77 47.75,49.78 47.75,53.59 49.53,56.9 69.09,56.9 70.36,55.63 10.ORDER_FILTER_CURRENT.1
SIGNAL_I_4
  Bottom 0.406: A/D-CONVERTER.6 89.41,40.39 91.44,42.93 91.44,48.51 90.42,49.28 85.34,49.28 84.84,49.78 84.84,51.31 85.34,51.82 88.65,51.82 89.66,53.09 89.66,54.61 88.65,55.63 76.71,55.63 75.18,53.85 75.18,42.93 73.91,41.91 10.ORDER_FILTER_CURRENT.8
SIGNAL_U_0
  Bottom 0.406: 90.17,81.92 REED_RELAIS_.P$4 | T_R2.1 T_R1.2
  Bottom 0.61: T_R2.1 89.15,90.42 90.17,89.41 | 90.17,89.41 90.17,81.92 | VOLTAGE_INPUT.1 92.71,91.95 90.17,89.41
SIGNAL_U_1
  Bottom 0.406: T_D1.A 106.05,81.79 | 106.05,81.79 T_R12.2 | 106.05,81.79 108.2,81.79 | 108.2,81.79 T_D2.C | VOLTAGE-FOLLOWER_VOLTAGE.3 132.59,72.64 133.35,71.88 133.35,66.55 132.08,65.53 115.32,65.53 113.28,67.31 109.22,67.31 108.2,68.33 108.2,81.79
SIGNAL_U_2
  Bottom 0.406: VOLTAGE-FOLLOWER_VOLTAGE.2 128.02,70.1 126.49,72.64 | 126.49,72.64 VOLTAGE-FOLLOWER_VOLTAGE.6 | PGA_VOLTAGE.10 125.22,82.8 126.49,81.28 126.49,72.64
SIGNAL_U_3  (via drill 0.8)
  Top 0.406: v120.65,90.42 v120.65,53.34
  Bottom 0.406: v120.65,90.42 PGA_VOLTAGE.7 | v120.65,53.34 121.92,52.07 10.ORDER_FILTER_VOLTAGE.1
SIGNAL_U_4
  Bottom 0.406: 10.ORDER_FILTER_VOLTAGE.8 131.83,53.59 131.06,54.1 122.68,54.1 118.87,58.67 94.23,58.67 89.92,50.55 A/D-CONVERTER.2
SPICS0
  Bottom 0.406: A/D-CONVERTER.14 99.06,53.09 96.01,47.75 96.01,35.31 97.54,33.02 97.54,12.7 98.3,11.94 110.74,11.94 111.51,12.7 PI_CONNECTION.24
SPIMISO
  Bottom 0.406: A/D-CONVERTER.11 100.08,44.7 99.31,43.94 99.31,37.34 102.62,33.27 102.62,19.05 103.12,18.54 107.19,18.54 107.7,19.05 107.7,20.83 108.46,21.59 112.52,21.59 PI_CONNECTION.21
SPISCLK
  Bottom 0.406: A/D-CONVERTER.13 100.08,50.55 97.54,46.99 97.54,36.32 100.08,33.27 100.08,13.72 100.58,13.21 109.73,13.21 110.24,13.72 110.24,18.8 111.25,19.81 PI_CONNECTION.23
V_REF  (via drill 0.8)
  Top 0.406: v83.31,64.52 v83.31,53.09
  Bottom 0.406: CURRENT_SEN..3 22.1,47.75 26.42,43.18 32.77,43.18 35.05,44.96 PGA_CURRENT.9 38.86,44.96 39.62,44.2 39.62,40.13 47.75,30.99 R_C2.1 51.56,30.99 53.59,29.46 REFERENC_VOLTAGE.6 57.91,29.46 58.67,30.23 58.67,32.51 59.69,33.78 68.58,33.78 69.34,34.54 69.34,38.1 70.61,39.37 74.93,39.37 78.99,42.93 81.28,42.93 | PGA_VOLTAGE.9 123.44,85.09 126.49,85.09 128.52,82.8 | 128.52,82.8 PGA_VOLTAGE.1 | v83.31,64.52 105.92,64.52 107.44,66.04 111.25,66.04 113.28,64.01 132.84,64.01 134.87,65.53 134.87,73.15 134.11,73.91 128.78,73.91 128.52,74.17 128.52,82.8 | 81.28,48.26 A_C2.1 81.28,42.93 | 81.28,48.26 A_C1.1 81.28,52.32 82.04,53.09 v83.31,53.09 A/D-CONVERTER.1 | A/D-CONVERTER.3 86.87,48.26 81.28,48.26 | A/D-CONVERTER.5 81.28,42.93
